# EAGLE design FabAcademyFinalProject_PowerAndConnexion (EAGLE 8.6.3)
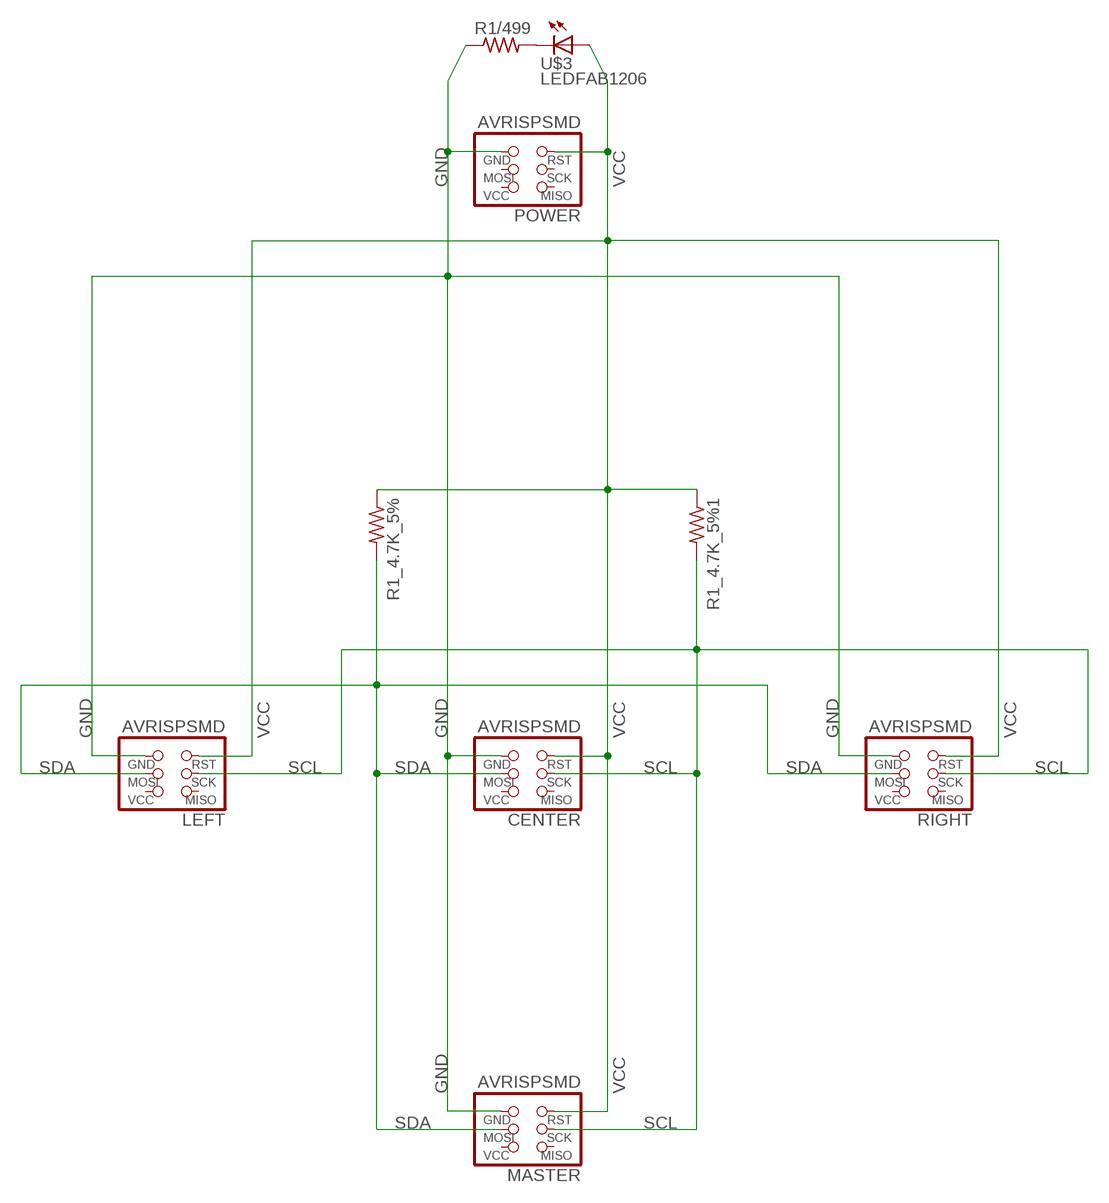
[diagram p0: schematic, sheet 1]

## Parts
CENTER  AVRISPSMD  [2X03SMD]
LEFT  AVRISPSMD  [2X03SMD]
MASTER  AVRISPSMD  [2X03SMD]
POWER  AVRISPSMD  [2X03SMD]
R1/499  RES-US1206FAB  [R1206FAB]
R1_4.7K_5%  RES-US1206FAB  [R1206FAB]
R1_4.7K_5%1  RES-US1206FAB  [R1206FAB]
RIGHT  AVRISPSMD  [2X03SMD]
U$3  LEDFAB1206  [LED1206FAB]

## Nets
GND: CENTER.6(GND) LEFT.6(GND) MASTER.6(GND) POWER.6(GND) R1/499.1 RIGHT.6(GND)
N$2: R1/499.2 U$3.2(C)
SCL: CENTER.3(SCK) LEFT.3(SCK) MASTER.3(SCK) R1_4.7K_5%1.2 RIGHT.3(SCK)
SDA: CENTER.4(MOSI) LEFT.4(MOSI) MASTER.4(MOSI) R1_4.7K_5%.2 RIGHT.4(MOSI)
VCC: CENTER.5(RST) LEFT.5(RST) MASTER.5(RST) POWER.5(RST) R1_4.7K_5%1.1 R1_4.7K_5%.1 RIGHT.5(RST) U$3.1(A)
Unconnected: CENTER.1(MISO) CENTER.2(VCC) LEFT.1(MISO) LEFT.2(VCC) MASTER.1(MISO) MASTER.2(VCC) POWER.1(MISO) POWER.2(VCC) POWER.3(SCK) POWER.4(MOSI) RIGHT.1(MISO) RIGHT.2(VCC)

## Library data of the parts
CENTER LEFT MASTER POWER RIGHT = fab:AVRISP
R1/499 R1_4.7K_5% R1_4.7K_5%1 = fab:RES-US: Resistor (US Symbol)
U$3 = fab:LED: LED

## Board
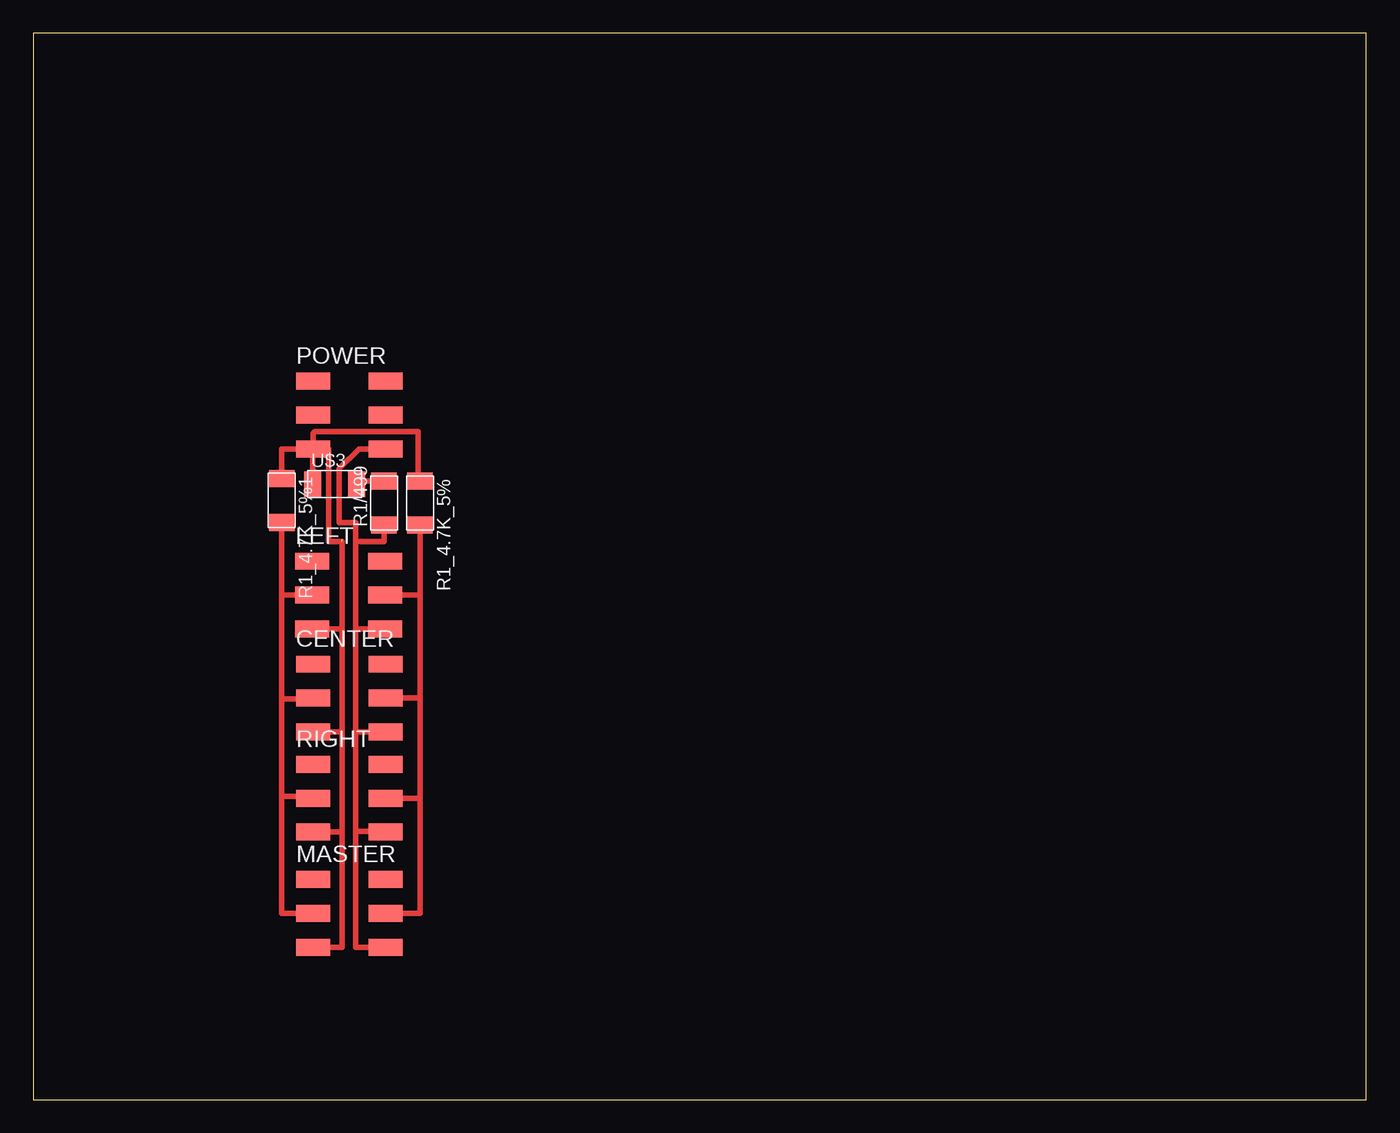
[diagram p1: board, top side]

Size 100 x 80 mm. Coordinates in mm from the lower left corner, seen from the top.
Outline: 0,0 100,0 100,80 0,80 0,0
Copper layers (1*16): Top 0.035mm / dielectric 1.5mm / Bottom 0.035mm
Design rules "default *": minimum track width 6mil, minimum drill 0.35mm, track to track 16mil, track to pad 16mil, pad to pad 16mil, via to via 16mil, smd to smd 16mil, copper to edge 40mil, drill to drill 6mil, minimum pad ring 10mil, minimum via ring 8mil, stop-mask expansion 4mil, vias tented up to drill 0mil, thermal gap 10mil

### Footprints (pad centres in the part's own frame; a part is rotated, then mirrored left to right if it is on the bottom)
2X03SMD = smd 2.54 x 1.27: 1 -2.54,2.54; 2 2.92,2.54; 3 -2.54,0; 4 2.92,0; 5 -2.54,-2.54; 6 2.92,-2.54
R1206FAB = smd 1.27 x 1.905: 1 -1.651,0; 2 1.651,0
LED1206FAB = smd 1.27 x 1.905: 1 -1.651,0; 2 1.651,0

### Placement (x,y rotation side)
CENTER  23.52,30.12 0 top
LEFT  23.47,37.85 0 top
MASTER  23.52,13.97 0 top
POWER  23.52,51.36 0 top
R1/499  26.31,44.75 90 top
R1_4.7K_5%  29.01,44.75 270 top
R1_4.7K_5%1  18.64,44.96 270 top
RIGHT  23.52,22.61 0 top
U$3  22.61,46.18 0 top

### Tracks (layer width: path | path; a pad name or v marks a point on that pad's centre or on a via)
GND
  Top 0.406: 24.18,35.31 24.18,27.58 | 24.18,27.58 24.18,20.12 | 24.18,20.12 26.44,20.12 RIGHT.6 | 24.18,20.12 24.18,11.43 MASTER.6 | 24.18,27.58 CENTER.6 | 24.18,35.31 LEFT.6 | POWER.6 24.45,48.82 22.96,47.33 22.96,43.28 24.18,43.28 24.18,41.86 | 24.18,35.31 24.18,41.86 | R1/499.1 26.31,41.86 24.18,41.86
N$2
  Top 0.406: U$3.2 24.26,46.41 R1/499.2
SCL
  Top 0.406: R1_4.7K_5%1.2 18.64,37.85 | 18.64,37.85 LEFT.3 | 18.64,37.85 18.64,30.07 | CENTER.3 20.98,30.07 18.64,30.07 | 18.64,30.07 18.64,22.96 18.64,22.76 | RIGHT.3 20.98,22.76 18.64,22.76 | 18.64,22.76 18.64,13.97 MASTER.3
SDA
  Top 0.406: R1_4.7K_5%.2 29.01,37.85 | 29.01,37.85 LEFT.4 | 29.01,37.85 29.01,30.12 | 29.01,30.12 CENTER.4 | 29.01,30.12 29.01,22.61 | 29.01,22.61 RIGHT.4 | 29.01,22.61 29.01,13.97 MASTER.4
VCC  (1 unrouted)
  Top 0.406: POWER.5 18.64,48.82 R1_4.7K_5%1.1 | POWER.5 20.98,49.96 21.13,50.11 28.85,50.11 28.85,46.41 R1_4.7K_5%.1 | 23.16,20.07 RIGHT.5 | 23.16,35.31 23.16,41.86 22.15,41.86 22.15,48.82 POWER.5 | 23.16,35.31 23.16,27.58 | 23.16,27.58 23.16,20.07 | 23.16,20.07 23.16,11.43 MASTER.5 | 23.16,27.58 CENTER.5 | 23.16,35.31 LEFT.5 | U$3.1 20.95,48.82 POWER.5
